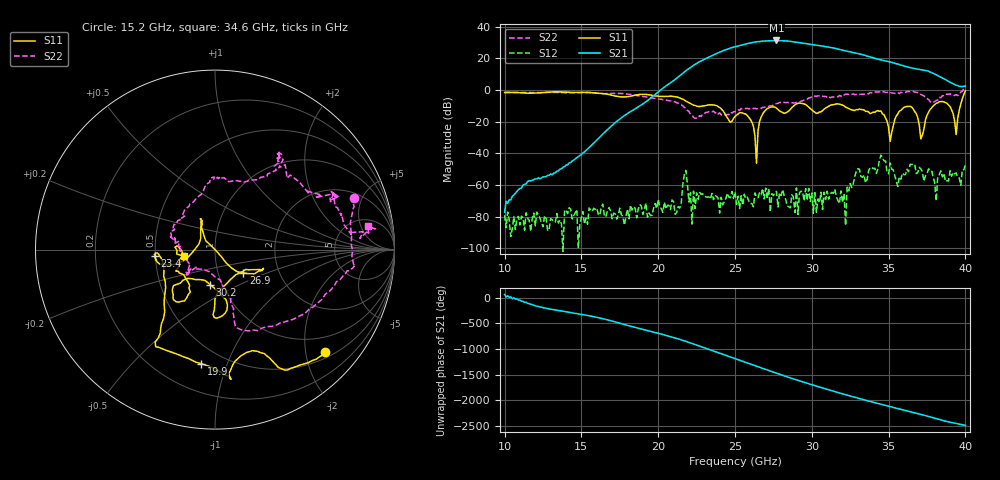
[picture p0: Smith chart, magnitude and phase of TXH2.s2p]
!Keysight Technologies,M9808A,MY58100618,A.14.70.03
!Date: Monday, February 27, 2023 13:18:15
!Correction: S11(C  2-Port  )
!S21(C  2-Port  )
!S12(C  2-Port  )
!S22(C  2-Port  )
!S2P File: Measurements: S11, S21, S12, S22:
# Hz S  RI  R 50
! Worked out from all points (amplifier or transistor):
!   301 points, 10 GHz to 40 GHz, reference 50 ohm
!   highest |S21| = 31.3 dB at 27.7 GHz (marker M1)
!   |S21| within 3 dB of that: 25.38 GHz to 30.27 GHz (4.883 GHz wide, 17.5 % of centre)
!   unconditionally stable (mu >= 1): start of sweep to 39.85 GHz
!   at 15 GHz: K = 54538.44, MAG = -30.5 dB, |S12| = -80.6 dB
!   at 25 GHz: K = 33.99, MAG = 27.5 dB, |S12| = -64.5 dB
!   at 40 GHz: K = -7.90, MSG = 24.9 dB, |S12| = -47.4 dB
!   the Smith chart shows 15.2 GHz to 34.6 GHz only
!   S11 on the Smith chart (normalised r, x): 15.2 GHz: 0.63, -2.40; 19.9 GHz: 0.38, -0.81; 23.4 GHz: 0.50, -0.04; 26.9 GHz: 1.32, -0.36; 30.2 GHz: 0.88, -0.36; 34.6 GHz: 0.71, -0.05
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1e10  0.7362 0.367  5.84e-05 0.000123  -9.88e-05 -4.67e-05  0.0228 0.8399
1.5e10  0.6393 -0.5469  0.00747 0.00537  1.07e-05 -9.31e-05  0.7665 0.3008
1.52e10  0.6137 -0.5697  0.00993 0.00483  4.77e-05 -3.25e-05  0.7733 0.2901
1.99e10  -0.0779 -0.6355  0.6277 0.4758  0.000149 -9.68e-05  0.3165 -0.4274
2e10  -0.1084 -0.6265  0.7578 0.4169  -0.000115 0.000326  0.2915 -0.4292
2.34e10  -0.3348 -0.037  5.28 10.21  0.000299 0.000186  -0.1605 -0.1258
2.43e10  -0.1831 -0.0656  15.3 -9.362  -6.4e-05 0.00028  -0.1576 -0.0587
2.5e10  -0.079 0.1221  -6.555 -22.09  -0.000467 0.000374  -0.201 0.0471
2.59e10  -0.0724 0.1145  -27.7 11.09  -0.000233 0.000197  -0.2246 0.1139
2.64e10  0.0033 -0.0035  -8.428 32.18  2.23e-05 0.000417  -0.1869 0.1696
2.69e10  0.1585 -0.1304  21.98 27.48  -0.000309 -0.000178  -0.146 0.2409
2.77e10  0.2421 -0.111  30.69 -19.88  -0.000582 0.000216  -0.0451 0.3659
2.83e10  0.0856 -0.1672  -2.778 -35.36  0.000251 0.00024  0.0172 0.3957
2.89e10  -0.0041 -0.337  -29.21 -14.17  -1.46e-05 0.000133  0.0903 0.3804
3e10  0.0202 -0.2357  -5.45 26.7  0.000552 1.76e-05  0.3619 0.4908
3.02e10  -0.0268 -0.1953  2.976 26.08  0.000567 -8.64e-06  0.3559 0.5287
3.1e10  -0.2106 -0.1925  22.61 4.295  -3.37e-05 -0.000629  0.3554 0.456
3.19e10  -0.1864 -0.2878  6.937 -17.2  0.000635 -8.03e-05  0.5581 0.2897
3.31e10  -0.2182 -0.1197  -13.42 -2.698  -0.00058 -0.00304  0.6826 0.2326
3.46e10  -0.1718 -0.0369  2.631 8.265  0.00538 0.00448  0.8522 0.1293
3.5e10  -0.0387 -0.0515  5.848 5.27  0.000116 -0.00222  0.7806 0.1238
4e10  0.4719 -0.8069  1.193 0.5754  -0.00358 0.00232  1.106 -0.7024
